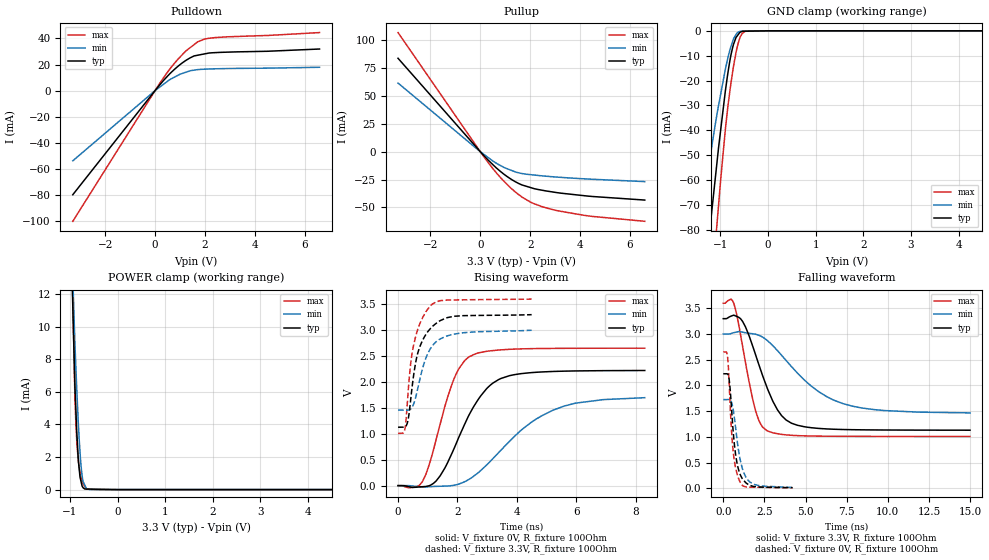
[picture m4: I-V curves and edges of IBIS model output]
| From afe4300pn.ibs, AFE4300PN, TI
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|   output Model
[Model]   output
Model_type   3-state
Polarity   Non-Inverting
Vmeas = 1.65
Vref = 1.65
Cref = 2pF
Rref = 50
|   typ   min   max
|   (nom PVT)   (fast PVT)   (slow PVT)
|C_comp from frequency sweep method (F=4MHz)
|C_comp   6.673e-12   5.997e-12   7.886e-12
|ON state : BUFFER OUTPUT TURNED HIGH
|C_comp   6.673e-12   5.997e-12   7.886e-12
|OFF state: BUFFER IN HIGH IMPEDANCE
|C_comp   3.857e-12   3.023e-12   4.721e-12
|C_comp from LC tank measurement(L=1nH)
|Resonant Frequency(Hz)   3.120e+09   3.480e+09   2.850e+09
 C_comp   2.605e-12   2.094e-12   3.122e-12
|ON state : BUFFER OUTPUT TURNED HIGH
|Resonant Frequency(Hz)   3.120e+09   3.480e+09   2.850e+09
|C_comp   2.605e-12   2.094e-12   3.122e-12
|OFF state: BUFFER IN HIGH IMPEDANCE
|Resonant Frequency(Hz)   3.200e+09   3.610e+09   2.890e+09
|C_comp   2.476e-12   1.946e-12   3.036e-12
| Where nom  PVT is Nominal Process, 3.3V, 27C
|   Fast PVT is Strong Process,  3.6V, 0C
|   Slow PVT is Weak Process,   3V, 70C
[Voltage Range]   3.3   3   3.6
|Ambient Temperature   25   70   0
|Junction Temperature
[Temperature Range]   27   70   0
[Pullup Reference]   3.3   3   3.6
[Pulldown Reference]   0   0   0
[Power Clamp Reference]   3.3   3   3.6
[GND Clamp Reference]   0   0   0
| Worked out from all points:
|   slope of the pulldown table from 0 to 0.495 V, typ, clamps not added: 45.2 ohm
|   slope of the pullup table from 0 to 0.495 V, typ, clamps not added: 43.4 ohm
|   GND clamp passes 1 mA (typ) near -0.61 V on its own axis
|   POWER clamp passes 1 mA (typ) near -0.80 V on its own axis
|   falling waveform, V_fixture 3.3V, R_fixture 100Ohm: 20-80 % time 1.55ns typ, 3.1ns min, 953ps max; typ from 3.3 V to 1.13 V
|   rising waveform, V_fixture 0V, R_fixture 100Ohm: 20-80 % time 1.18ns typ, 2ns min, 816ps max; typ from 0 V to 2.22 V
|   rising waveform, V_fixture 3.3V, R_fixture 100Ohm: 20-80 % time 475ps typ, 522ps min, 401ps max; typ from 1.13 V to 3.3 V
|   falling waveform, V_fixture 0V, R_fixture 100Ohm: 20-80 % time 406ps typ, 517ps min, 327ps max; typ from 2.23 V to 0.011 V
[Pulldown]
|   Voltage   I(typ)   I(min)   I(max)
-3.3V     -79.67mA   -53.72mA   -100mA
212.4mV   4.969mA    3.063mA    6.309mA
633.6mV   13.7mA     8.887mA    17.52mA
1.092V    21.23mA    13.17mA    27.51mA
1.399V    25.01mA    15.13mA    32.77mA
1.706V    27.1mA     16.09mA    37.32mA
2.012V    28.24mA    16.46mA    39.56mA
2.473V    29.16mA    16.75mA    40.71mA
6.6V      31.88mA    17.9mA     44.47mA
[GND Clamp]
|   Voltage   I(typ)   I(min)   I(max)
-3.3V     -521.3mA   -378.1mA   -651.2mA
-1.416V   -117.3mA   -76.78mA   -161.6mA
-1.211V   -77.77mA   -50.07mA   -110.6mA
-1.116V   -60.68mA   -38.48mA   -87.58mA
-1.065V   -51.53mA   -32.66mA   -75.89mA
-896.4mV  -24.13mA   -15.38mA   -39.54mA
-815.1mV  -13.46mA   -8.681mA   -26.15mA
-726mV    -5.448mA   -3.239mA   -14.34mA
-669.6mV  -2.594mA   -1.41mA    -8.359mA
-591mV    -607.7uA   -235.3uA   -2.792mA
-439.2mV  -145uA     -72uA      -75.42uA
6.6V      0A         0A         0A
[Pullup]
|   Voltage   I(typ)   I(min)   I(max)
-3.3V     83.82mA    61.59mA    106.9mA
183.6mV   -4.495mA   -3.078mA   -5.792mA
633.6mV   -14.37mA   -10.22mA   -18.7mA
939.6mV   -20.06mA   -13.99mA   -26.37mA
1.44V     -27.37mA   -18.44mA   -36.8mA
1.706V    -30.09mA   -19.74mA   -41.2mA
2.117V    -32.89mA   -20.86mA   -46.31mA
2.473V    -34.57mA   -21.69mA   -49.29mA
3.089V    -36.79mA   -22.83mA   -52.95mA
4.498V    -40.22mA   -24.77mA   -58.11mA
6.6V      -43.43mA   -26.86mA   -62.48mA
[POWER Clamp]
|   Voltage   I(typ)   I(min)   I(max)
-3.3V     258.7mA    230.6mA    287.2mA
-1.04V    22.32mA    21.98mA    25.15mA
-897.6mV  6.456mA    9.067mA    5.832mA
-878.4mV  5.051mA    7.66mA     4.25mA
-858mV    3.559mA    6.189mA    3.045mA
-835.2mV  2.374mA    4.722mA    2.101mA
-788.7mV  757.6uA    2.294mA    1.065mA
-771mV    536.5uA    1.57mA     780uA
-726mV    118.5uA    502.3uA    358.4uA
-689.7mV  35.58uA    276uA      199.1uA
-591mV    30.46uA    6.868uA    22.8uA
6.6V      0A         0A         0A
[Ramp]
R_load = 100
|   typ   min   max
dV/dt_r   1.33615/1.17882e-09   1.03268/2.04661e-09   1.59263/8.15529e-10
dV/dt_f   1.30255/1.54277e-09   0.920398/3.08993e-09   1.55558/9.52966e-10
[Falling Waveform]
V_fixture = 3.3V
V_fixture_min = 3V
V_fixture_max = 3.6V
R_fixture = 100Ohm
|   Time   V(typ)   V(min)   V(max)
0s        3.3V       3V         3.6V
648ps     3.367V     3.028V     3.588V
1.172ns   3.248V     3.037V     2.767V
1.894ns   2.665V     3.002V     1.592V
2.256ns   2.318V     2.964V     1.256V
2.674ns   1.947V     2.876V     1.117V
3.294ns   1.526V     2.679V     1.06V
4.142ns   1.266V     2.369V     1.03V
7.276ns   1.143V     1.647V     1.01V
15ns      1.129V     1.466V     1.007V
[Rising Waveform]
V_fixture = 0V
V_fixture_min = 0V
V_fixture_max = 0V
R_fixture = 100Ohm
|   Time   V(typ)   V(min)   V(max)
0s        1.537nV    1.828nV    1.416nV
830ps     -20.53mV   -28mV      87.22mV
1.292ns   96.6mV     -13.87mV   914.7mV
1.836ns   651mV      2.898mV    1.99V
2.406ns   1.381V     126.6mV    2.491V
2.974ns   1.866V     394mV      2.592V
3.384ns   2.046V     635.7mV    2.618V
4.178ns   2.164V     1.087V     2.64V
5.208ns   2.204V     1.454V     2.649V
8.306ns   2.223V     1.698V     2.653V
[Rising Waveform]
V_fixture = 3.3V
V_fixture_min = 3V
V_fixture_max = 3.6V
R_fixture = 100Ohm
|   Time   V(typ)   V(min)   V(max)
0s        1.128V     1.457V     1.007V
234ps     1.133V     1.457V     1.098V
318ps     1.218V     1.457V     1.631V
418ps     1.616V     1.475V     2.318V
580ps     2.333V     1.673V     2.848V
760ps     2.718V     2.118V     3.161V
1.084ns   3.028V     2.64V      3.466V
1.386ns   3.174V     2.82V      3.565V
1.896ns   3.269V     2.925V     3.584V
4.498ns   3.3V       2.999V     3.6V
[Falling Waveform]
V_fixture = 0V
V_fixture_min = 0V
V_fixture_max = 0V
R_fixture = 100Ohm
|   Time   V(typ)   V(min)   V(max)
0s        2.227V     1.725V     2.653V
234ps     2.227V     1.725V     2.61V
350ps     2.132V     1.725V     2.098V
466ps     1.723V     1.698V     1.304V
614ps     1.06V      1.509V     685.3mV
770ps     612.4mV    1.123V     369.5mV
1.022ns   271.1mV    566mV      120.7mV
1.372ns   106.5mV    217.3mV    25.16mV
1.858ns   32.81mV    76.11mV    21.04mV
4.214ns   11.34mV    16.96mV    6.873mV
